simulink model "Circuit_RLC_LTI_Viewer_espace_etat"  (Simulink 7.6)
settings: Solver=ode23tb  StartTime=0.0  StopTime=0.04  RelTol=1e-3
libraries: powerlib x14

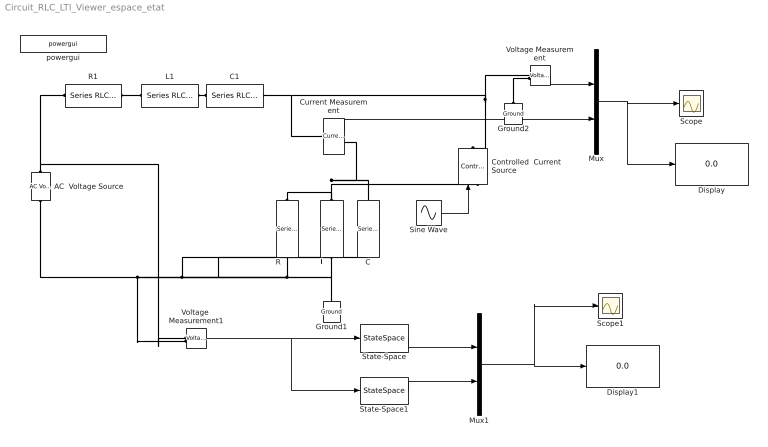
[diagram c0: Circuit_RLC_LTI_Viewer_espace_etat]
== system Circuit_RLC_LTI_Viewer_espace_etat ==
  AC  Voltage Source : powerlib/Electrical Sources/AC Voltage Source  DialogController=POWERSYS.PowerSysDialog  SystemSampleTime=-1  Amplitude=100  Phase=0  Frequency=60  SampleTime=0  Measurements=None
  C : powerlib/Elements/Series RLC Branch  DialogController=POWERSYS.PowerSysDialog  PhysicalDomain=powersysdomain  SubClassName=unknown  LeftPortType=p1  RightPortType=p1  LConnTagsString=__new0  RConnTagsString=__new0  BranchType=C  Resistance=1  Inductance=1e-3  SetiL0=off  InitialCurrent=0  Capacitance=0.001  Setx0=off  InitialVoltage=0  Measurements=None
  C1 : powerlib/Elements/Series RLC Branch  DialogController=POWERSYS.PowerSysDialog  PhysicalDomain=powersysdomain  SubClassName=unknown  LeftPortType=p1  RightPortType=p1  LConnTagsString=__new0  RConnTagsString=__new0  BranchType=C  Resistance=1  Inductance=1e-3  SetiL0=off  InitialCurrent=0  Capacitance=0.001  Setx0=off  InitialVoltage=0  Measurements=None
  Controlled  Current Source : powerlib/Electrical Sources/Controlled Current Source  DialogController=POWERSYS.PowerSysDialog  SystemSampleTime=-1  Initialize=on  Source_Type=AC  Amplitude=0  Phase=0  Frequency=0  Measurements=None
  Current Measurement : powerlib/Measurements/Current Measurement  DialogController=POWERSYS.PowerSysDialog  SystemSampleTime=-1  PhasorSimulation=off  OutputType=Complex  PSBequivalent=0
  Display : Display
  Display1 : Display
  Ground1 : powerlib/Elements/Ground  DialogController=POWERSYS.PowerSysDialog  PhysicalDomain=powersysdomain  SubClassName=unknown  LeftPortType=p1  RightPortType=p1  LConnTagsString=a
  Ground2 : powerlib/Elements/Ground  DialogController=POWERSYS.PowerSysDialog  PhysicalDomain=powersysdomain  SubClassName=unknown  LeftPortType=p1  RightPortType=p1  LConnTagsString=a
  L : powerlib/Elements/Series RLC Branch  DialogController=POWERSYS.PowerSysDialog  PhysicalDomain=powersysdomain  SubClassName=unknown  LeftPortType=p1  RightPortType=p1  LConnTagsString=__new0  RConnTagsString=__new0  BranchType=L  Resistance=4  Inductance=10e-3  SetiL0=off  InitialCurrent=0  Capacitance=0  Setx0=off  InitialVoltage=0  Measurements=None
  L1 : powerlib/Elements/Series RLC Branch  DialogController=POWERSYS.PowerSysDialog  PhysicalDomain=powersysdomain  SubClassName=unknown  LeftPortType=p1  RightPortType=p1  LConnTagsString=__new0  RConnTagsString=__new0  BranchType=L  Resistance=4  Inductance=10e-3  SetiL0=off  InitialCurrent=0  Capacitance=0  Setx0=off  InitialVoltage=0  Measurements=None
  Mux : Mux  Inputs=2
  Mux1 : Mux  Inputs=2
  R : powerlib/Elements/Series RLC Branch  DialogController=POWERSYS.PowerSysDialog  PhysicalDomain=powersysdomain  SubClassName=unknown  LeftPortType=p1  RightPortType=p1  LConnTagsString=__new0  RConnTagsString=__new0  BranchType=R  Resistance=4  Inductance=10e-3  SetiL0=off  InitialCurrent=0  Capacitance=0  Setx0=off  InitialVoltage=0  Measurements=None
  R1 : powerlib/Elements/Series RLC Branch  DialogController=POWERSYS.PowerSysDialog  PhysicalDomain=powersysdomain  SubClassName=unknown  LeftPortType=p1  RightPortType=p1  LConnTagsString=__new0  RConnTagsString=__new0  BranchType=R  Resistance=4  Inductance=10e-3  SetiL0=off  InitialCurrent=0  Capacitance=0  Setx0=off  InitialVoltage=0  Measurements=None
  Scope : Scope
  Scope1 : Scope
  Sine Wave : Sin  Frequency=10  SampleTime=0
  State-Space : StateSpace  A=|  B=|  C="[1\t0\t0\t0 ]"  D=0
      | [-250,0,-1000,-1000
      | ;0,0,0,1000; 100,0,0,0
      | ; 100,-100,0,-400
      | ]
      | [0;
      | 0;
      | 0;-100]
  State-Space1 : StateSpace  A=|  B=|  C="[0\t0\t0\t-1 ]"  D=0
      | [-250	0	-1000	-1000; 0	0	0	1000;100	0	0	0
      | ;100	-100	0	-400
      | ]
      | [0;
      | 0;
      | 0;
      | -100]
  Voltage  Measurement1 : powerlib/Measurements/Voltage Measurement  DialogController=POWERSYS.PowerSysDialog  SystemSampleTime=-1  PhasorSimulation=off  OutputType=Complex  PSBequivalent=0
  Voltage Measurement : powerlib/Measurements/Voltage Measurement  DialogController=POWERSYS.PowerSysDialog  SystemSampleTime=-1  PhasorSimulation=off  OutputType=Complex  PSBequivalent=0
  powergui : powerlib/powergui  Priority=1  SystemSampleTime=-1  SimulationMode=Continuous  SampleTime=50e-6  frequency=60  SPID=off  DisableSnubberDevices=off  DisableRonSwitches=off  DisableVfSwitches=off  SwTol=0  Interpol=off  frequencyindice=0  echomessages=off  HookPort=off  DisplayEquations=off  FunctionMessages=off  EnableUseOfTLC=off  x0status=blocks  RestoreLinks=warning  ResistiveCurrentMeasurement=off  Frange=[0:2:500]  Ylog=off  Xlog=on  ShowGrid=on  save=off  variable=ZData  ZoomFFT=off  StartTime=0.0  cycles=1  DisplayStyle=1  fundamental=60  FreqAxis=off  MaxFrequency=1000  frequencyindicesteady=1  display=off  methode=off
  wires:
  Mux/1 -> Scope/1, Display/1
  Voltage Measurement/1 -> Mux/1
  Current Measurement/1 -> Mux/2
  Sine Wave/1 -> Controlled  Current Source/1
  Voltage  Measurement1/1 -> State-Space/1, State-Space1/1
  State-Space/1 -> Mux1/1
  State-Space1/1 -> Mux1/2
  Mux1/1 -> Display1/1, Scope1/1
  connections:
  R/LConn1 -- L/RConn1 -- Ground1/LConn1 -- C/RConn1 -- Controlled  Current Source/LConn1 -- AC  Voltage Source/LConn1 -- Voltage  Measurement1/LConn2
  Current Measurement/LConn1 -- Voltage Measurement/LConn1 -- Controlled  Current Source/RConn1 -- C1/LConn1
  R1/RConn1 -- L1/RConn1
  AC  Voltage Source/RConn1 -- R1/LConn1 -- Voltage  Measurement1/LConn1
  Ground2/LConn1 -- Voltage Measurement/LConn2
  R/RConn1 -- C/LConn1 -- Current Measurement/RConn1 -- L/LConn1
  L1/LConn1 -- C1/RConn1
